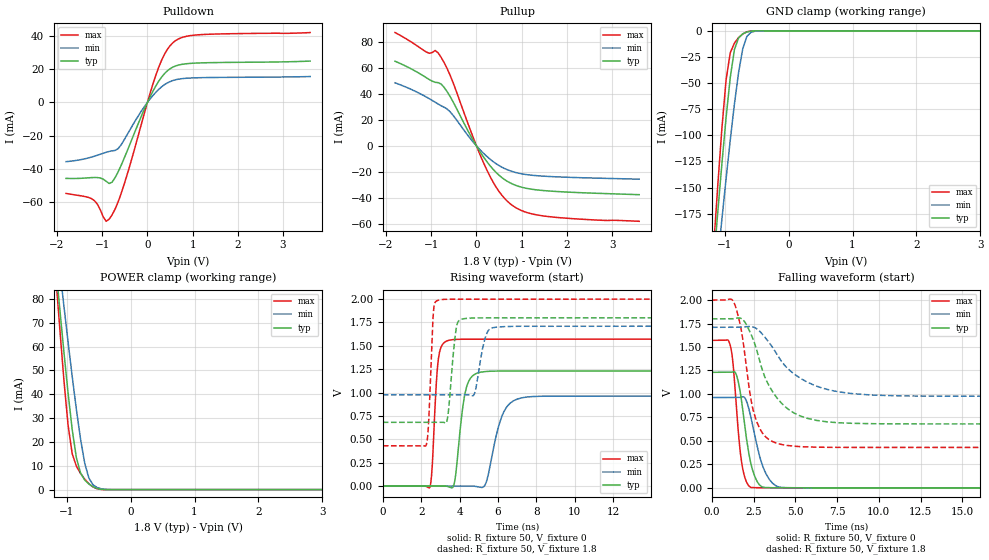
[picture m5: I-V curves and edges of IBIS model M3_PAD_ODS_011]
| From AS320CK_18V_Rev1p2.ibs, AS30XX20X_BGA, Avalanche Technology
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[Model] M3_PAD_ODS_011
Model_type I/O
Enable   Active-High
Vinl  =  0.63
Vinh  =  1.17
Vmeas =  0.9
Cref  =  30e-12
| Capacitance  typ   min   max
C_comp   1.624629e-12   1.520611e-12   1.744819e-12
| Variables   typ   min   max
[GND Clamp Reference]   0   0   0
[POWER Clamp Reference]   1.8   1.71   2
[Pulldown Reference]   0   0   0
[Pullup Reference]   1.8   1.71   2
[Temperature Range]   25   125   -40
[Voltage Range]   1.8   1.71   2
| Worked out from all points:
|   slope of the pulldown table from 0 to 0.27 V, typ, clamps not added: 20 ohm
|   slope of the pullup table from 0 to 0.27 V, typ, clamps not added: 19.4 ohm
|   GND clamp passes 1 mA (typ) near -0.64 V on its own axis
|   POWER clamp passes 1 mA (typ) near -0.57 V on its own axis
|   falling waveform, R_fixture 50, V_fixture 0: 20-80 % time 622ps typ, 820ps min, 446ps max; typ from 1.23 V to 0 V
|   falling waveform, R_fixture 50, V_fixture 1.8: 20-80 % time 1.67ns typ, 2.4ns min, 856ps max; typ from 1.8 V to 0.681 V
|   rising waveform, R_fixture 50, V_fixture 0: 20-80 % time 414ps typ, 685ps min, 242ps max; typ from 0 V to 1.23 V
|   rising waveform, R_fixture 50, V_fixture 1.8: 20-80 % time 286ps typ, 389ps min, 186ps max; typ from 0.681 V to 1.8 V
[GND Clamp]
| Voltage   I(typ)   I(min)   I(max)
-1.8V     -720.4mA   -670.5mA   -825.2mA
-1.173V   -222.3mA   -260.3mA   -207.5mA
-1.108V   -173.8mA   -219.8mA   -148.3mA
-1.043V   -126.9mA   -180.1mA   -93.11mA
-977.6mV  -83.02mA   -141.5mA   -47.01mA
-912.4mV  -44.68mA   -104.6mA   -21.04mA
-847.2mV  -17.95mA   -70.1mA    -11.75mA
-782.1mV  -6.736mA   -39.85mA   -6.526mA
-716.9mV  -2.917mA   -17.13mA   -2.96mA
-651.7mV  -1.107mA   -5.246mA   -907.6uA
-456.2mV  -3.886uA   -74.14uA   -373.5nA
3.6V      0A         0A         0A
[POWER Clamp]
| Voltage   I(typ)   I(min)   I(max)
-1.8V     287.1mA    268.3mA    329.6mA
-1.173V   94.89mA    108.5mA    91.02mA
-1.108V   76.1mA     92.66mA    67.97mA
-1.043V   57.9mA     77.16mA    46.14mA
-977.6mV  40.62mA    62.05mA    27.14mA
-912.4mV  25.13mA    47.46mA    15.06mA
-847.2mV  13.38mA    33.64mA    9.853mA
-716.9mV  4.014mA    11.09mA    4.394mA
-651.7mV  2.34mA     4.821mA    2.483mA
-586.6mV  1.18mA     2.003mA    1.113mA
-325.9mV  1.153uA    19.85uA    110.1nA
3.6V      0A         0A         0A
[Pulldown]
| Voltage   I(typ)   I(min)   I(max)
-1.8V     -45.66mA   -35.6mA    -54.71mA
-1.238V   -45.19mA   -32.87mA   -57.82mA
-912.4mV  -47.39mA   -29.98mA   -71.44mA
-847.2mV  -48.72mA   -29.47mA   -70.19mA
-716.9mV  -45.32mA   -28.86mA   -64.22mA
-521.4mV  -34.04mA   -22.82mA   -49.79mA
-65.17mV  -3.915mA   -2.451mA   -6.278mA
248.3mV   12.65mA    7.772mA    20.97mA
434.5mV   18.83mA    11.62mA    31.58mA
620.7mV   21.87mA    13.59mA    37.09mA
1.179V    23.74mA    14.86mA    40.71mA
3.6V      24.84mA    15.54mA    41.96mA
[Pullup]
| Voltage   I(typ)   I(min)   I(max)
-1.8V     65.14mA    48.52mA    87.22mA
-1.108V   52.47mA    37.59mA    72.25mA
-912.4mV  48.92mA    33.58mA    73.42mA
-782.1mV  47.58mA    30.91mA    68.21mA
-586.6mV  38.24mA    26.39mA    54.73mA
-65.17mV  3.89mA     2.658mA    5.836mA
248.3mV   -12.95mA   -8.678mA   -19.85mA
496.6mV   -22.51mA   -15.08mA   -34.96mA
744.8mV   -28.48mA   -19.19mA   -44.52mA
1.055V    -32.3mA    -21.85mA   -50.58mA
1.49V     -34.42mA   -23.33mA   -53.98mA
3.6V      -37.57mA   -25.63mA   -58.07mA
[Ramp]
dV/dt_r   0.738287/0.413697n  0.577195/0.685288n  0.942684/0.241691n
dV/dt_f   0.67144/1.67235n  0.440569/2.39751n  0.941874/0.855767n
R_load = 50
[Falling Waveform]
R_fixture = 50
V_fixture = 0
V_fixture_min = 0
V_fixture_max = 0
| Time   V(typ)   V(min)   V(max)
0s        1.23V      962mV      1.571V
1.112ns   1.231V     962.2mV    1.51V
1.274ns   1.235V     962.2mV    1.313V
1.462ns   1.206V     962.3mV    877.3mV
1.776ns   928.3mV    967.1mV    278mV
2.059ns   542.1mV    930.2mV    66.95mV
2.359ns   242.4mV    734.3mV    3.158mV
3.063ns   8.393mV    223mV      712.7uV
3.974ns   997uV      11.56mV    677.1uV
21.88ns   263.8nV    1.563uV    204.5nV
[Falling Waveform]
R_fixture = 50
V_fixture = 1.8
V_fixture_min = 1.71
V_fixture_max = 2
| Time   V(typ)   V(min)   V(max)
0s        1.8V       1.71V      2V
1.372ns   1.805V     1.711V     1.954V
1.75ns    1.805V     1.711V     1.691V
2.284ns   1.66V      1.718V     1.001V
2.543ns   1.546V     1.709V     782.8mV
3.157ns   1.187V     1.609V     555.7mV
3.812ns   978.5mV    1.447V     479.5mV
5.362ns   761.5mV    1.161V     438.4mV
8.041ns   689.9mV    1.012V     430.9mV
21.88ns   680.9mV    975.7mV    430.2mV
[Rising Waveform]
R_fixture = 50
V_fixture = 0
V_fixture_min = 0
V_fixture_max = 0
| Time   V(typ)   V(min)   V(max)
0s        1.762nV    42.9nV     1.422nV
2.441ns   -526.4uV   -424.5uV   -16.49mV
2.891ns   -623.6uV   -502.8uV   1.358V
3.322ns   -2.781mV   -577.7uV   1.552V
3.712ns   19.48mV    -645.5uV   1.568V
4.283ns   993.6mV    -744.8uV   1.571V
4.909ns   1.208V     -8.195mV   1.571V
6.295ns   1.23V      790.5mV    1.571V
7.215ns   1.23V      942.4mV    1.571V
21.88ns   1.23V      962mV      1.571V
[Rising Waveform]
R_fixture = 50
V_fixture = 1.8
V_fixture_min = 1.71
V_fixture_max = 2
| Time   V(typ)   V(min)   V(max)
0s        680.9mV    975.7mV    430.2mV
2.251ns   681.6mV    976.2mV    434.6mV
2.636ns   681.7mV    976.3mV    1.868V
2.847ns   681.8mV    976.4mV    1.986V
3.341ns   696.5mV    976.5mV    1.999V
3.813ns   1.675V     976.6mV    1.999V
4.083ns   1.784V     976.6mV    1.999V
4.758ns   1.798V     981.3mV    1.999V
5.706ns   1.799V     1.693V     1.999V
21.88ns   1.8V       1.71V      2V
